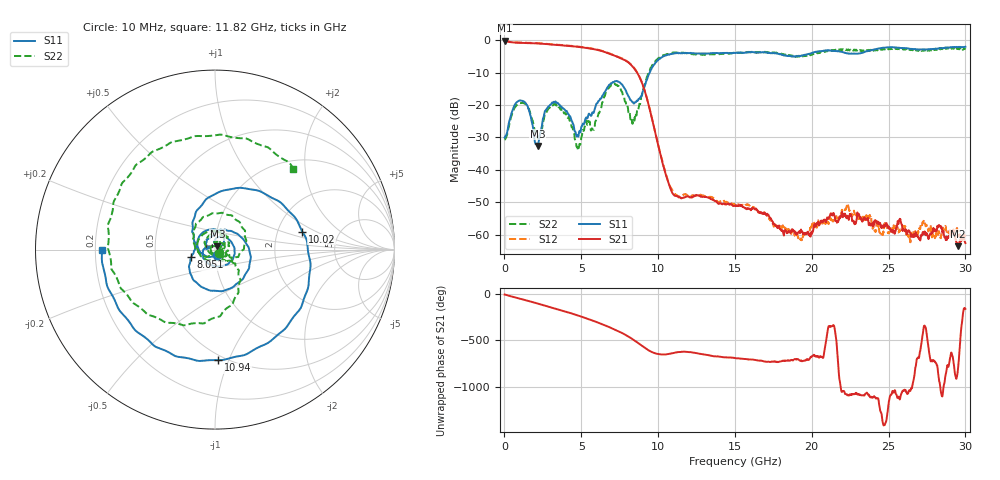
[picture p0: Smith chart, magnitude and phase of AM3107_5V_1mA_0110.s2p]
# Hz S DB R 50.0
!freq dBS11 angS11 dBS21 angS21 dBS12 angS12 dBS22 angS22
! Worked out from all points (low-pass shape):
!   1601 points, 10 MHz to 30 GHz, reference 50 ohm
!   highest |S21| = -0.22 dB at 10 MHz (marker M1); lowest = -63.6 dB at 29.49 GHz (marker M2)
!   |S21| within 3 dB of the highest: start of sweep to 6.217 GHz
!   lowest |S11| = -32.6 dB at 2.166 GHz (marker M3), VSWR 1.05, Z = 51.3 + j1.96 ohm
!   |S11| at or under -10 dB: start of sweep to 9.449 GHz
!   |S22| runs from -34.0 to -2.3 dB; largest |S21 - S12| = 0.013
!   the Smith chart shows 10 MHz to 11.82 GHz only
!   S11 on the Smith chart (normalised r, x): 10 MHz: 1.02, -0.06; 8.051 GHz: 0.76, -0.07; 10.02 GHz: 2.75, +0.73; 10.94 GHz: 0.46, -0.92; 11.82 GHz: 0.23, -0.00
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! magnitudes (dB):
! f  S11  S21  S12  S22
! 10 MHz  -30.1  -0.2  -0.1  -30.7
! 1.116 GHz  -18.7  -0.9  -0.8  -19.4
! 2.166 GHz  -32.6  -1.0  -0.9  -30.2
! 2.653 GHz  -21.8  -1.2  -1.1  -22.9
! 3.196 GHz  -19.1  -1.4  -1.3  -19.8
! 4.171 GHz  -22.9  -1.8  -1.7  -23.7
! 4.733 GHz  -29.4  -2.1  -2.0  -32.8
! 5.015 GHz  -26.6  -2.2  -2.1  -29.8
! 6.964 GHz  -13.3  -4.4  -4.3  -13.8
! 8.051 GHz  -17.2  -6.8  -6.8  -21.8
! 8.463 GHz  -19.4  -8.8  -8.7  -24.8
! 10.02 GHz  -6.1  -32.6  -32.6  -5.6
! 10.94 GHz  -4.2  -47.2  -46.4  -3.8
! 11.82 GHz  -4.0  -48.3  -47.7  -4.0
! 15.01 GHz  -3.9  -51.1  -50.8  -3.9
! 19.24 GHz  -4.9  -59.1  -61.3  -4.8
! 20.01 GHz  -4.0  -59.0  -57.0  -4.5
! 22.26 GHz  -4.1  -54.9  -51.5  -2.9
! 25.01 GHz  -2.2  -57.5  -59.6  -2.8
! 28.33 GHz  -2.5  -57.5  -60.4  -2.5
! 29.49 GHz  -2.1  -63.6  -58.7  -2.7
! 30 GHz  -2.0  -62.6  -59.1  -2.5
